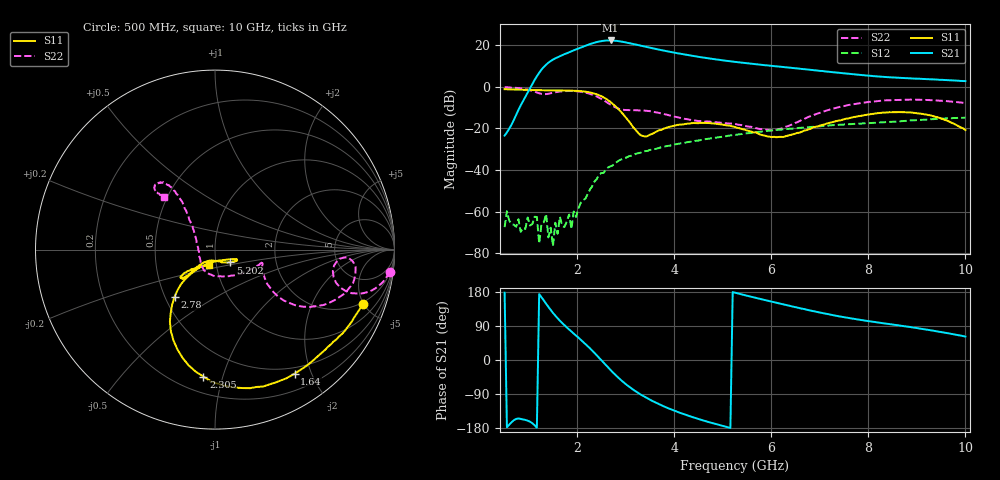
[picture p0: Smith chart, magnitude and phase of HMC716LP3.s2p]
! Chelmsford, MA 01824
! http://www.hittite.com
! Tel: 978-250-3343
! Fax: 978-250-3373
! Device  :  HMC716LP3
! Description:  GaAs PHEMT MMIC LOW NOISE AMPLIFIER
! Frequency  :  3.1-3.9 GHz
! Package  :  LP3  - 3x3 mm Quad Flatpack No-Lead (QFN) Plastic Package: 16 pin
! Ports  :  2 RF, 2 DC
!  Pin  2  = Rfin  = Port 1
!  Pin  11 = Rfout = Port 2
!  Pin  15 = vdd
! Voltages:  VDD  = 5.0 Volts
! Rbias  :  Rbias  = 820 OHMS
! Currents :  Idd  = 75.0 mA
! Data:  The device was measured on evaluation board 122540-1.
!  Data was collected using a calibrated network analyzer.The DC block was removed in the input port.
!  The evaluation circuit board was modeled and simulated.  This was use
!  to removed the evaluation board circuit from the measured data.
!  The reference plane is the center of the package pin.
! Misc:  Lot #
!Date Measured:  10 - 24 -2008
!Date:  10 - 24 -2008 LHS
!Date:  2010-03-17  MJV file corrected for control line.
! Note:
!  Hittite Microwave supplies this data as a sample of measured data at the
!  package pin for this package product.  Your particular data for this product
!  may vary.
!  Data was taken at 25 degrees C.
!  Hittite Microwave reserves the right to change this data at anytime.
# MHz S  MA  R 50
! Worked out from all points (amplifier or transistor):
!   201 points, 500 MHz to 10 GHz, reference 50 ohm
!   highest |S21| = 22.3 dB at 2.685 GHz (marker M1)
!   |S21| within 3 dB of that: 2.117 GHz to 3.402 GHz (1.285 GHz wide, 46.6 % of centre)
!   unconditionally stable (mu >= 1): start of sweep to end of sweep
!   at 2.067 GHz: K = 6.17, MAG = 26.4 dB, |S12| = -55.7 dB
!   at 5.25 GHz: K = 1.90, MAG = 12.1 dB, |S12| = -23.1 dB
!   at 10 GHz: K = 1.80, MAG = 3.6 dB, |S12| = -14.8 dB
!   S11 on the Smith chart (normalised r, x): 500 MHz: 1.83, -4.91; 1.64 GHz: 0.41, -1.76; 2.305 GHz: 0.30, -0.87; 2.78 GHz: 0.56, -0.33; 5.202 GHz: 1.17, -0.17; 10 GHz: 0.92, -0.16
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500  0.8786 -20.3  0.06737 177.5  0.0004279 119.8  0.9826 -7.2
927.5  0.8499 -33.4  0.5741 -158.1  0.0003858 114.4  0.8813 -15.6
1165  0.8305 -40.6  1.792 -178.5  0.0007496 43.3  0.7294 -16.9
1212.5  0.8296 -42.2  2.172 174.0  0.0001736 -53.4  0.6992 -15.3
1402.5  0.8247 -48.4  3.786 140.2  0.0002422 -151.1  0.6808 -5.7
1640  0.8212 -57.3  5.434 103.7  0.0007574 -74.9  0.7696 -4.8
1877.5  0.8101 -67.9  7.133 75.3  0.0003857 16.0  0.794 -11.6
2115  0.777 -81.5  9.173 48.4  0.001881 -7.7  0.7435 -20.7
2305  0.7105 -95.2  11.02 25.0  0.004097 -11.1  0.6493 -29.0
2495  0.5944 -110.6  12.5 -0.6  0.0085 -30.6  0.5117 -35.6
2685  0.4318 -124.9  12.98 -26.5  0.01232 -52.9  0.3741 -34.7
2780  0.3458 -130.6  12.77 -38.7  0.0148 -63.2  0.3227 -30.2
2922.5  0.2347 -135.2  12.12 -55.6  0.01825 -74.9  0.2832 -21.8
3112.5  0.1241 -129.5  10.93 -74.9  0.02214 -91.3  0.2745 -14.4
3397.5  0.06414 -76.5  9.218 -98.1  0.02863 -110.1  0.2677 -16.1
3682.5  0.0904 -38.1  7.8 -116.7  0.03406 -123.5  0.2366 -26.4
4205  0.1272 -24.5  5.993 -143.3  0.0453 -143.8  0.1706 -58.0
5202.5  0.1118 -40.0  4.037 179.2  0.06867 -171.4  0.1312 -118.0
5250  0.108 -41.0  3.976 177.6  0.07015 -172.6  0.1283 -120.1
6865  0.1068 -133.0  2.518 128.8  0.1093 151.1  0.2087 131.3
8432.5  0.2452 -138.7  1.697 94.8  0.1431 122.9  0.4738 128.3
10000  0.09174 -112.3  1.372 61.8  0.1823 94.8  0.4089 133.8
